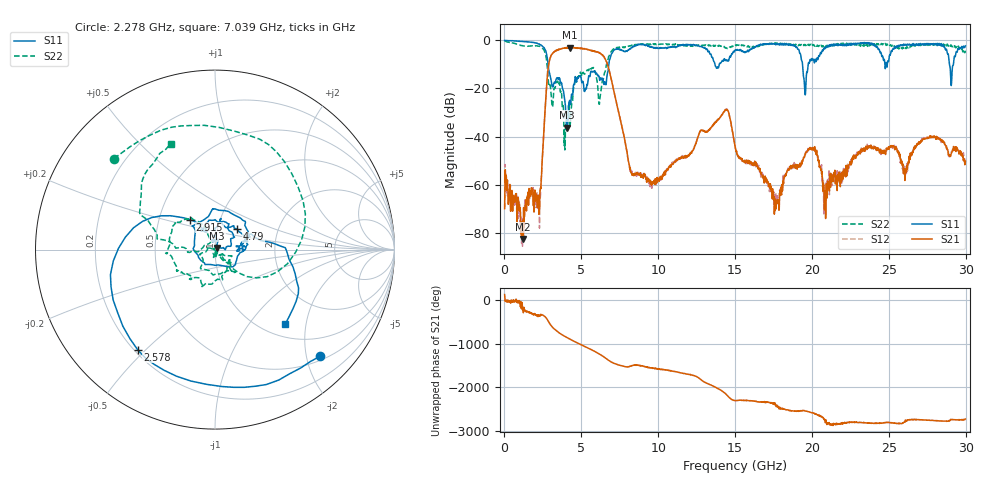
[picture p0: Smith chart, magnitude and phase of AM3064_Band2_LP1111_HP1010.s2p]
# Hz S DB R 50.0
!freq dBS11 angS11 dBS21 angS21 dBS12 angS12 dBS22 angS22
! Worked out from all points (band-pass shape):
!   1600 points, 10 MHz to 29.98 GHz, reference 50 ohm
!   highest |S21| = -2.98 dB at 4.246 GHz (marker M1); lowest = -82.6 dB at 1.21 GHz (marker M2)
!   |S21| within 3 dB of the highest: 3.065 GHz to 6.338 GHz (3.273 GHz wide, 69.6 % of centre)
!   lowest |S11| = -36.3 dB at 4.04 GHz (marker M3), VSWR 1.03, Z = 51.3 + j0.917 ohm
!   |S11| at or under -10 dB: 2.838 GHz to 6.785 GHz (3.946 GHz wide, 82 % of centre); 19.39 GHz to 19.76 GHz (369.8 MHz wide, 1.89 % of centre); 28.94 GHz to 29.2 GHz (256.5 MHz wide, 0.882 % of centre)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
!   |S22| runs from -45.6 to -0.1 dB; largest |S21 - S12| = 0.019
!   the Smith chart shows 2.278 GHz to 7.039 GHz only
!   S11 on the Smith chart (normalised r, x): 2.278 GHz: 0.58, -2.27; 2.578 GHz: 0.21, -0.47; 2.915 GHz: 0.72, +0.25; 4.79 GHz: 1.25, +0.29; 7.039 GHz: 1.24, -1.53
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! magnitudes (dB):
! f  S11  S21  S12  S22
! 10 MHz  0.0  -70.0  -69.8  -0.1
! 1.21 GHz  -0.5  -82.6  -74.2  -2.3
! 2.278 GHz  -1.6  -70.3  -78.1  -2.4
! 2.578 GHz  -3.0  -36.1  -36.0  -4.1
! 2.915 GHz  -13.2  -8.7  -8.6  -18.9
! 3.553 GHz  -15.7  -3.9  -3.7  -17.7
! 4.04 GHz  -36.3  -3.2  -3.0  -35.5
! 4.246 GHz  -24.9  -3.0  -3.1  -34.9
! 4.79 GHz  -15.5  -3.2  -3.1  -15.6
! 5.015 GHz  -17.0  -3.5  -3.4  -14.6
! 6.214 GHz  -16.4  -5.4  -5.2  -24.0
! 7.039 GHz  -4.9  -18.8  -18.8  -3.9
! 8.276 GHz  -2.9  -55.2  -54.2  -2.0
! 10 GHz  -3.3  -58.0  -58.2  -1.6
! 14.37 GHz  -8.4  -28.8  -28.8  -3.3
! 15 GHz  -4.1  -44.4  -44.0  -2.1
! 17.7 GHz  -1.4  -66.8  -67.2  -1.5
! 19.56 GHz  -22.7  -47.3  -46.9  -1.8
! 19.99 GHz  -7.6  -45.1  -44.9  -1.6
! 20.83 GHz  -3.6  -62.6  -66.1  -2.3
! 25 GHz  -8.4  -44.6  -44.5  -1.6
! 29.98 GHz  -2.3  -50.3  -51.4  -4.3
